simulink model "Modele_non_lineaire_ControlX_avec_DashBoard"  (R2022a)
settings: Solver=ode3  StartTime=0.0  StopTime=inf  FixedStep=dt  RelTol=1e-3  EnableMultiTasking=on
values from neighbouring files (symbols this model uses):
  B = 4    [param.m]
  fw = fv*R^2/i^2    (= 0.00135235635389)    [param.m]
  i = 3    [param.m]
  Jeq = meq*(R/i)^2    (= 0.000216377016623)    [param.m]
  kc = 0.21    [param.m]
  ke = 0.2083    [param.m]
  L = 3.2e-3    (= 0.0032)    [param.m]
  r = 5.1    [param.m]
  R = 155/(2*pi)/1000    (= 0.0246690161792)    [param.m]
  Vsat = 10    [param.m]
undefined symbols (not defined in the file or in its folder): sigbuilder_block
libraries: simulink x2

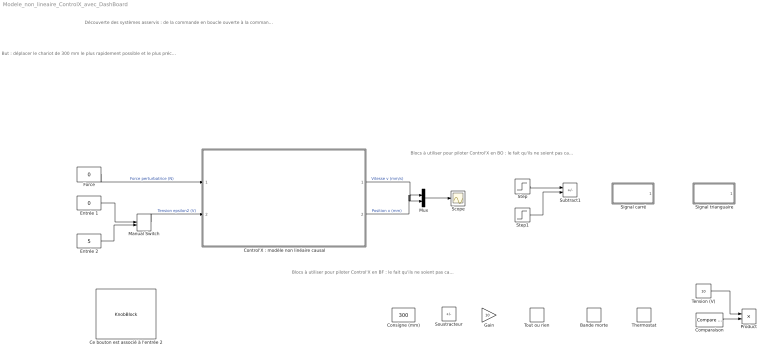
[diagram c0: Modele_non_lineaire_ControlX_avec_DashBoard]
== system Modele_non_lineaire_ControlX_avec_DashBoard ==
  note: Découverte des systèmes asservis : de la commande en boucle ouverte à la commande en boucle fermée
  note: Blocs à utiliser pour piloter Control'X en BF : le fait qu'ils ne soient pas cablés ne gène pas la simulation
  note: But : déplacer le chariot de 300 mm le plus rapidement possible et le plus précisemment possible Lancer le script "param.m" Lancer une simulation : la durée de simulation est infinie, la case "Enable pacing to slow done the simulation" est cochée, elle se trouve dans "Simulation Pacing" sous le bouton "Run" Observer les courbes de simulation Basculer l'interrupteur "Manual switch" Modifier éventuellement les valeurs numériques des entrées Changer éventuellement de stratégie de pilotage, Changer éventuellement la durée de simulation (autour de 0.5 s par exemple pour les stratégies de pilotage en boucle fermée par exemple)
  note: Blocs à utiliser pour piloter Control'X en BO : le fait qu'ils ne soient pas cablés ne gène pas la simulation
  Bande morte : DeadZone  LowerValue=-1  UpperValue=1
  Ce bouton est associé à l'entrée 2 : KnobBlock  ScaleMin=-10  ScaleMax=10
  Comparaison : simulink/Logic and Bit Operations/Compare To Constant  relop=<=  const=300  OutDataTypeStr=boolean
  Consigne (mm) : Constant  Value=300
  "Control'X : modèle non linéaire causal" : Subsystem
  Entrée 1 : Constant  Value=0
  Entrée 2 : Constant  Value=5
  Force : Constant  Value=0
  Gain : Gain  Gain=10
  Manual Switch : ManualSwitch
  Mux : Mux  Inputs=2
  Product : Product
  Scope : Scope
  Signal carré : Subsystem  Tag=STV Subsys  LoadFcn=sigbuilder_block('load');  StartFcn=sigbuilder_block('start');  StopFcn=sigbuilder_block('stop');  ClipboardFcn=sigbuilder_block('clipboard');  mask(Sigbuilder block){tuvar=[0:10]}
      mask help: Simulink:masks:SigbuilderBlock_MD
      mask init:
      | if ~strcmp(get_param(bdroot(gcbh),'SimulationStatus'),'stopped') tuvar = sigbuilder_block('maskInit'); end
  Signal trianguaire : Subsystem  Tag=STV Subsys  LoadFcn=sigbuilder_block('load');  StartFcn=sigbuilder_block('start');  StopFcn=sigbuilder_block('stop');  ClipboardFcn=sigbuilder_block('clipboard');  mask(Sigbuilder block){tuvar=[0:10]}
      mask help: Simulink:masks:SigbuilderBlock_MD
      mask init:
      | if ~strcmp(get_param(bdroot(gcbh),'SimulationStatus'),'stopped') tuvar = sigbuilder_block('maskInit'); end
  Soustracteur : Sum  Inputs=+-
  Step : Step  After=10  SampleTime=0
  Step1 : Step  Time=2  After=10  SampleTime=0
  Subtract1 : Sum  Inputs=+-
  Tension (V) : Constant  Value=10
  Thermostat : Relay  OnSwitchValue=10  OffSwitchValue=10  OnOutputValue=10  OffOutputValue=-10
  Tout ou rien : Signum
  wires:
  Entrée 1/1 -> Manual Switch/1
  Entrée 2/1 -> Manual Switch/2
  Mux/1 -> Scope/1
  Manual Switch/1 -> "Control'X : modèle non linéaire causal"/2(Epsilon 2 (V))  "Tension epsilon2 (V)"
  Comparaison/1 -> Product/2
  Tension (V)/1 -> Product/1
  Force/1 -> "Control'X : modèle non linéaire causal"/1(Force perturbatrice (N))  "Force perturbatrice (N)"
  Step/1 -> Subtract1/1
  Step1/1 -> Subtract1/2
  "Control'X : modèle non linéaire causal"/1(Vitesse chariot (mm/s)) -> Mux/1  "Vitesse v (mm/s)"
  "Control'X : modèle non linéaire causal"/2(Position chariot (mm)) -> Mux/2  "Position x (mm)"

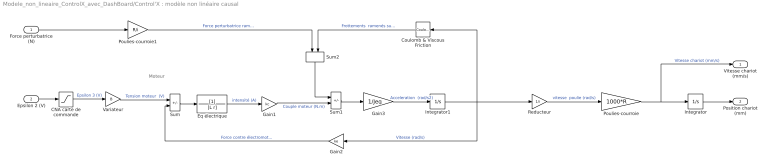
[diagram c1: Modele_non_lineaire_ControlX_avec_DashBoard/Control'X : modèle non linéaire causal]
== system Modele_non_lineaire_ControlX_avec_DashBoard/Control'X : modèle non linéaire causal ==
  note: Moteur
  Force perturbatrice (N) : Inport
  Epsilon 2 (V) : Inport  Port=2
  CNA carte de commande : Saturate  UpperLimit=Vsat  LowerLimit=-Vsat
  Coulomb & Viscous Friction : simulink/Discontinuities/Coulomb & Viscous Friction  offset=Cfrott  gain=fw
  Eq électrique : TransferFcn  Denominator=[L r]
  Gain1 : Gain  Gain=kc
  Gain2 : Gain  Gain=ke
  Gain3 : Gain  Gain=1/Jeq
  Integrator : Integrator
  Integrator1 : Integrator
  Poulies-courroie : Gain  Gain=1000*R
  Poulies-courroie1 : Gain  Gain=R/i
  Reducteur : Gain  Gain=1/i
  Sum : Sum  Inputs=+-
  Sum1 : Sum  Inputs=-+
  Sum2 : Sum
  Variateur : Gain  Gain=B
  Vitesse chariot (mm/s) : Outport
  Position chariot (mm) : Outport  Port=2
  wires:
  Coulomb & Viscous Friction/1 -> Sum2/2  "Frottements  ramenés sur le moteur (N.m)"
  Epsilon 2 (V)/1 -> CNA carte de commande/1
  CNA carte de commande/1 -> Variateur/1  "Epsilon 3 (V)"
  Eq électrique/1 -> Gain1/1  "intensité (A)"
  Variateur/1 -> Sum/1  "Tension moteur  (V)"
  Gain3/1 -> Integrator1/1  "Acceleration  (rad/s2)"
  Integrator1/1 -> Reducteur/1, Coulomb & Viscous Friction/1, Gain2/1  "Vitesse (rad/s)"
  Sum/1 -> Eq électrique/1
  Gain2/1 -> Sum/2  "Force contre électromotrice (V)"
  Gain1/1 -> Sum1/2  "Couple moteur (N.m)"
  Sum1/1 -> Gain3/1
  Poulies-courroie/1 -> Vitesse chariot (mm/s)/1, Integrator/1  "Vitesse chariot (mm/s)"
  Reducteur/1 -> Poulies-courroie/1  "vitesse  poulie (rad/s)"
  Sum2/1 -> Sum1/1
  Force perturbatrice (N)/1 -> Poulies-courroie1/1
  Integrator/1 -> Position chariot (mm)/1
  Poulies-courroie1/1 -> Sum2/1  "Force perturbatrice ramenée sur le moteur (N.m)"

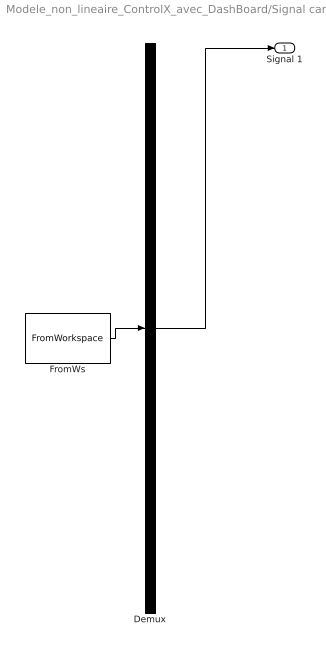
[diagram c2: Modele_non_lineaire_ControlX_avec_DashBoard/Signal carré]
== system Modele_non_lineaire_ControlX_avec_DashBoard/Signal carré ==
  Demux : Demux  Tag=STV Demux  Outputs=1
  FromWs : FromWorkspace  Tag=STV FromWs  VariableName=tuvar
  Signal 1 : Outport  Tag=STV Outport
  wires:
  Demux/1 -> Signal 1/1
  FromWs/1 -> Demux/1

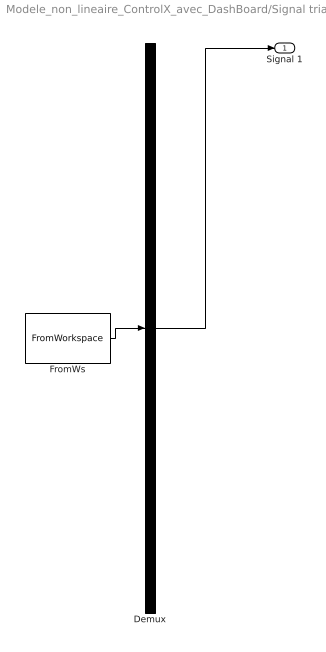
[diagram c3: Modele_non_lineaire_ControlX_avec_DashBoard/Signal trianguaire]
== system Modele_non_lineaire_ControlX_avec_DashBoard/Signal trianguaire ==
  Demux : Demux  Tag=STV Demux  Outputs=1
  FromWs : FromWorkspace  Tag=STV FromWs  VariableName=tuvar
  Signal 1 : Outport  Tag=STV Outport
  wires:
  FromWs/1 -> Demux/1
  Demux/1 -> Signal 1/1
